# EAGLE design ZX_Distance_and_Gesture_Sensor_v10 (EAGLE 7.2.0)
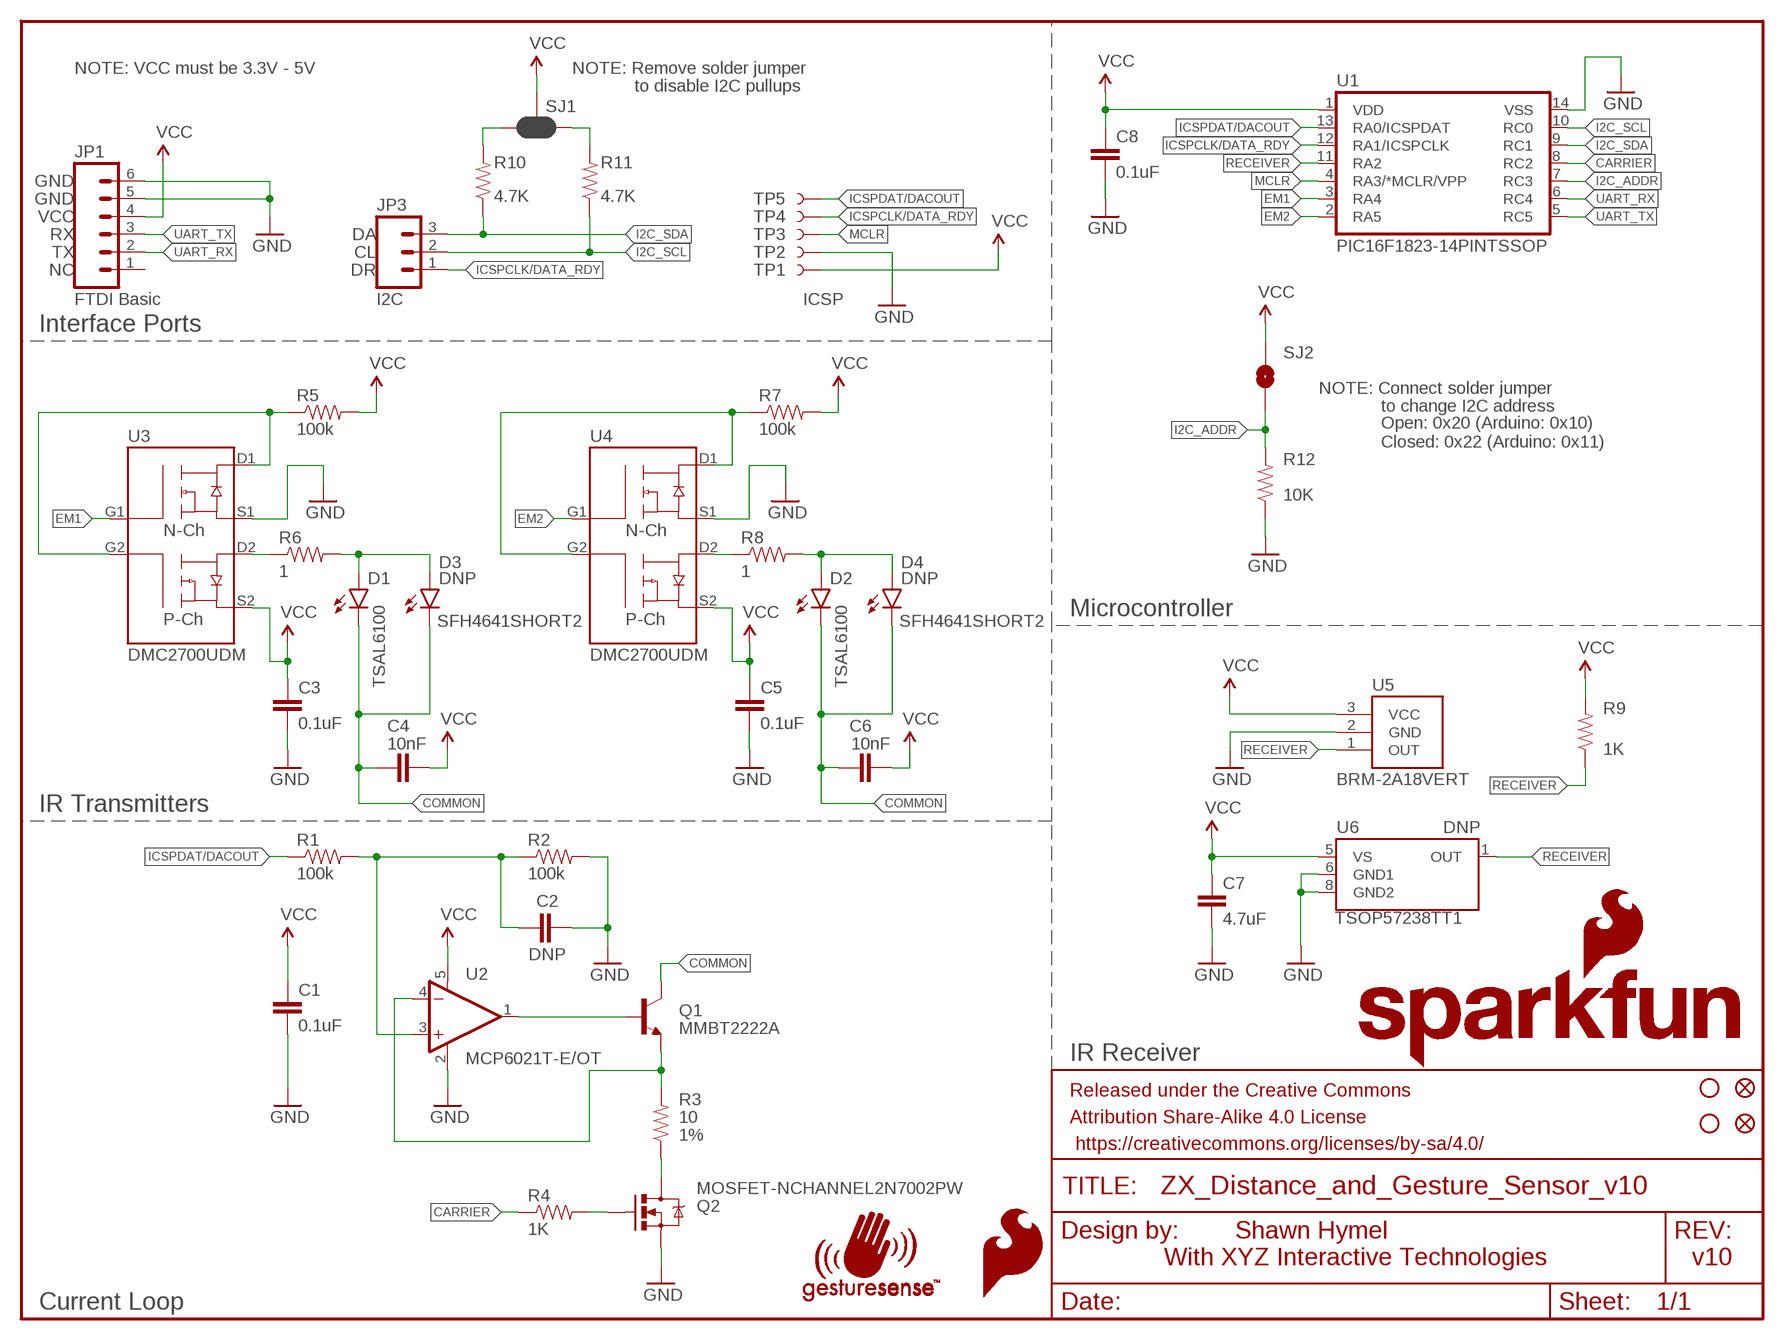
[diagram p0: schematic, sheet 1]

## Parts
C1  0.1uF  0.1UF-25V(+80/-20%)(0603)  [0603-CAP]
C2  DNP  CAP0603-CAP  [0603-CAP]
C3  0.1uF  0.1UF-25V(+80/-20%)(0603)  [0603-CAP]
C4  10nF  10NF/10000PF-50V-10%(0603)  [0603-CAP]
C5  0.1uF  0.1UF-25V(+80/-20%)(0603)  [0603-CAP]
C6  10nF  10NF/10000PF-50V-10%(0603)  [0603-CAP]
C7  4.7uF  4.7UF-6.3V-10%(0603)0603  [0603-CAP]
C8  0.1uF  0.1UF-25V(+80/-20%)(0603)  [0603-CAP]
D1  LED-IR-THRUTSAL6100  [LED5MM]
D2  LED-IR-THRUTSAL6100  [LED5MM]
D3  SFH4641SHORT2  [SFH4641-SHORT2]
D4  SFH4641SHORT2  [SFH4641-SHORT2]
FID1  FIDUCIAL1X2  [FIDUCIAL-1X2]
FID2  FIDUCIAL1X2  [FIDUCIAL-1X2]
FRAME1  FRAME-LETTER  [CREATIVE_COMMONS]
JP1  M06NO_SILK_FEMALE_PTH  [1X06_NO_SILK]
JP3  M031X03_NO_SILK  [1X03_NO_SILK]
LOGO1  SFE_LOGO_FLAME.1_INCH  [SFE_LOGO_FLAME_.1]
Q1  MMBT2222A  TRANSISTOR_NPNMMBT2222A  [SOT23-3]
Q2  MOSFET-NCHANNEL2N7002PW  [SOT323]
R1  100k  100KOHM-1/10W-1%(0603)  [0603-RES]
R2  100k  100KOHM-1/10W-1%(0603)  [0603-RES]
R3  10  10OHM-1/10W-1%(0603)SMD  [0603-RES]
R4  1K  1KOHM-1/10W-1%(0603)  [0603-RES]
R5  100k  100KOHM-1/10W-1%(0603)  [0603-RES]
R6  1  1OHM1/10W1%(0603)  [0603-RES]
R7  100k  100KOHM-1/10W-1%(0603)  [0603-RES]
R8  1  1OHM1/10W1%(0603)  [0603-RES]
R9  1K  1KOHM-1/10W-1%(0603)  [0603-RES]
R10  4.7K  4.7KOHM-1/10W-1%(0603)  [0603-RES]
R11  4.7K  4.7KOHM-1/10W-1%(0603)  [0603-RES]
R12  10K  10KOHM-1/10W-1%(0603)0603  [0603-RES]
SJ1  JUMPER-PAD-3-NC_BY_PASTE  [PAD-JUMPER-3-NC_BY_PASTE_YES_SILK_FULL_BOX]
SJ2  JUMPER-PAD-2-NOYES_SILK  [PAD-JUMPER-2-NO_YES_SILK]
STANDOFF1  STAND-OFF  [STAND-OFF]
STANDOFF2  STAND-OFF  [STAND-OFF]
TP1  TEST-POINT3X4  [PAD.03X.04]
TP2  TEST-POINT3X4  [PAD.03X.04]
TP3  TEST-POINT3X4  [PAD.03X.04]
TP4  TEST-POINT3X4  [PAD.03X.04]
TP5  TEST-POINT3X4  [PAD.03X.04]
U1  PIC16F1823-14PINTSSOP  [TSSOP14]
U2  MCP6021T-E/OT  [SOT23-5]
U3  DMC2700UDM  [SOT26]
U4  DMC2700UDM  [SOT26]
U5  BRM-2A18VERT  [BRM-2508_VERT]
U6  TSOP57238TT1  [TSOP572]
U$5  SFE_LOGO_NAME_FLAME.1_INCH  [SFE_LOGO_NAME_FLAME_.1]
U$6  GESTURESENSE_LOGOSTEXT  [GESTURESENSE_TEXT]

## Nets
CARRIER: R4.1 U1.8(RC2)
COMMON: C4.1 C6.1 D1.K(C) D2.K(C) D3.C D4.C Q1.3(C)
EM1: U1.3(RA4) U3.G1
EM2: U1.2(RA5) U4.G1
GND: C1.2 C2.2 C3.2 C5.2 C7.2 C8.2 JP1.5 JP1.6 Q2.2(S) R2.2 R12.1 TP2.P$1 U1.14(VSS) U2.2(V-) U3.S1 U4.S1 U5.2(GND) U6.6(GND1) U6.8(GND2)
I2C_ADDR: R12.2 SJ2.1 U1.7(RC3)
I2C_SCL: JP3.2 R11.1 U1.10(RC0)
I2C_SDA: JP3.3 R10.1 U1.9(RC1)
ICSPCLK/DATA_RDY: JP3.1 TP4.P$1 U1.12(RA1/ICSPCLK)
ICSPDAT/DACOUT: R1.1 TP5.P$1 U1.13(RA0/ICSPDAT)
MCLR: TP3.P$1 U1.4(RA3/*MCLR/VPP)
N$1: C2.1 R1.2 R2.1 U2.3(+IN)
N$2: Q1.2(E) R3.2 U2.4(-IN)
N$3: Q1.1(B) U2.1(OUT)
N$4: Q2.3(D) R3.1
N$5: Q2.1(G) R4.2
N$6: R6.1 U3.D2
N$7: D1.A D3.A R6.2
N$8: R5.1 U3.D1 U3.G2
N$9: R7.1 U4.D1 U4.G2
N$10: R10.2 SJ1.3
N$11: R8.1 U4.D2
N$12: D2.A D4.A R8.2
N$13: R11.2 SJ1.1
RECEIVER: R9.1 U1.11(RA2) U5.1(OUT) U6.1(OUT)
UART_RX: JP1.2 U1.6(RC4)
UART_TX: JP1.3 U1.5(RC5)
VCC: C1.1 C3.1 C4.2 C5.1 C6.2 C7.1 C8.1 JP1.4 R5.2 R7.2 R9.2 SJ1.2 SJ2.2 TP1.P$1 U1.1(VDD) U2.5(V+) U3.S2 U4.S2 U5.3(VCC) U6.5(VS)
Unconnected: JP1.1

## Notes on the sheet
- NOTE: VCC must be 3.3V - 5V | NOTE: Remove solder jumper
- to disable I2C pullups
- GND
- GND
- VCC
- RX | DA
- TX | CL
- NC | DR
- FTDI Basic | I2C | ICSP
- Interface Ports
- NOTE: Connect solder jumper
- to change I2C address
- Open: 0x20 (Arduino: 0x10)
  Closed: 0x22 (Arduino: 0x11)
- DNP | DNP
- Microcontroller
- IR Transmitters
- IR Receiver
- With XYZ Interactive Technologies
- Current Loop

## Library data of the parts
C1 C3 C5 C8 = SparkFun-Capacitors:0.1UF-25V(+80/-20%)(0603): CAP-00810; PROD_ID: CAP-00810
C2 = SparkFun-Capacitors:CAP: Capacitor
C4 C6 = SparkFun-Capacitors:10NF/10000PF-50V-10%(0603): CAP-00867; PROD_ID: CAP-00867
C7 = SparkFun-Capacitors:4.7UF-6.3V-10%(0603): CAP-08280; PROD_ID: CAP-08280
D1 D2 = SparkFun-LED:LED-IR-THRU; PROD_ID: DIO-12058; VARIANT: TSAL6100
D3 D4 = SparkFun-LED:SFH4641; PROD_ID: DIO-11994
FID1 FID2 = SparkFun-Aesthetics:FIDUCIAL: Fiducial Alignment Points
FRAME1 = SparkFun-Aesthetics:FRAME-LETTER: Schematic Frame; DESIGNER: Shawn Hymel; VERSION: v10
JP1 = SparkFun-Connectors:M06: Header 6 Standard 6-pin 0.1" header. Use with straight break away headers (SKU : PRT-00116), right angle break away headers (PRT-00553), swiss pins (PRT-00743), machine pins (PRT-00117), and female headers (PRT-00115). Molex polarized connector foot print use with SKU : PRT-08094 with associated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; PROD_ID: CONN-08437
JP3 = SparkFun-Connectors:M03: Header 3 Standard 3-pin 0.1" header. Use with straight break away headers (SKU : PRT-00116), right angle break away headers (PRT-00553), swiss pins (PRT-00743), machine pins (PRT-00117), and female headers (PRT-00115). Molex polarized connector foot print use with SKU : PRT-08232 with associated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
LOGO1 = SparkFun-Aesthetics:SFE_LOGO_FLAME: SFE Logo, flame only
Q1 = SparkFun-DiscreteSemi:TRANSISTOR_NPN: Generic NPN BJT MMBT2222A - TRANS-08049 (SOT-23, 1A 40V) MPSA42 - TRANS-09116 (SOT-23, 500mA 300V) MMBT5088LT1G - TRANS-11160 (SOT-23, 50 mA 30V) BC547 - COM-08928 (TO-92 45V 100mA) (1.Collector 2.Base 3.Emitter) 2N3904 - COM-00521 (TO-92 40V 200mA) (1.Emitter 2.Base 3.Collector) P2N2222A -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; PROD_ID: TRANS-08049
Q2 = SparkFun-DiscreteSemi:MOSFET-NCHANNEL: Common NMOSFET Parts MFG P/NStore IDProd ID FDD8780TRANS-09984 SI7820DNTRANS-11055 FDS6630AIC-08089 2N7002PWTRANS-11151 FQP30N06L COM-10213TRANS-10060 BSS123LT1GTRANS-08345 BSS138TRANS-00830 BS170 2N7000; PROD_ID: TRANS-11151
R1 R2 R5 R7 = SparkFun-Resistors:100KOHM-1/10W-1%(0603): RES-07828; PROD_ID: RES-07828
R3 = SparkFun-Resistors:10OHM-1/10W-1%(0603): RES-12581; PROD_ID: RES-12581; TOL: 1%
R4 R9 = SparkFun-Resistors:1KOHM-1/10W-1%(0603): RES-07856; PROD_ID: RES-07856
R6 R8 = SparkFun-Resistors:1OHM1/10W1%(0603): RES-08269; PROD_ID: RES-08269
R10 R11 = SparkFun-Resistors:4.7KOHM-1/10W-1%(0603): RES-07857; PROD_ID: RES-07857
R12 = SparkFun-Resistors:10KOHM-1/10W-1%(0603): RES-00824; PROD_ID: RES-00824
SJ1 = SparkFun-Passives:JUMPER-PAD-3-NC_BY_PASTE
SJ2 = SparkFun-Passives:JUMPER-PAD-2-NO
STANDOFF1 STANDOFF2 = SparkFun-Electromechanical:STAND-OFF: #4 Stand Off
TP1-TP5 = SparkFun-Passives:TEST-POINT: Bare copper test points for troubleshooting or ICT
U1 = SparkFun-DigitalIC:PIC16F1823-14PIN; PROD_ID: IC-11992
U2 = SparkFun-AnalogIC:MCP6021: Rail-to-rail input/output op-amp with 10 MHz bandwidth.; PROD_ID: IC-12504
U3 U4 = SparkFun-DiscreteSemi:DMC2700UDM; PROD_ID: TRANS-11993
U5 = SparkFun-Sensors:BRM-2A18: BRM-2A18 IR receiver.; PROD_ID: COMP-12505
U6 = SparkFun-Sensors:TSOP57238TT1; PLACE: DNP; PROD_ID: COMP-11990
U$5 = SparkFun-Aesthetics:SFE_LOGO_NAME_FLAME: SFE Logo, name and flame
U$6 = SparkFun-Aesthetics:GESTURESENSE_LOGOS

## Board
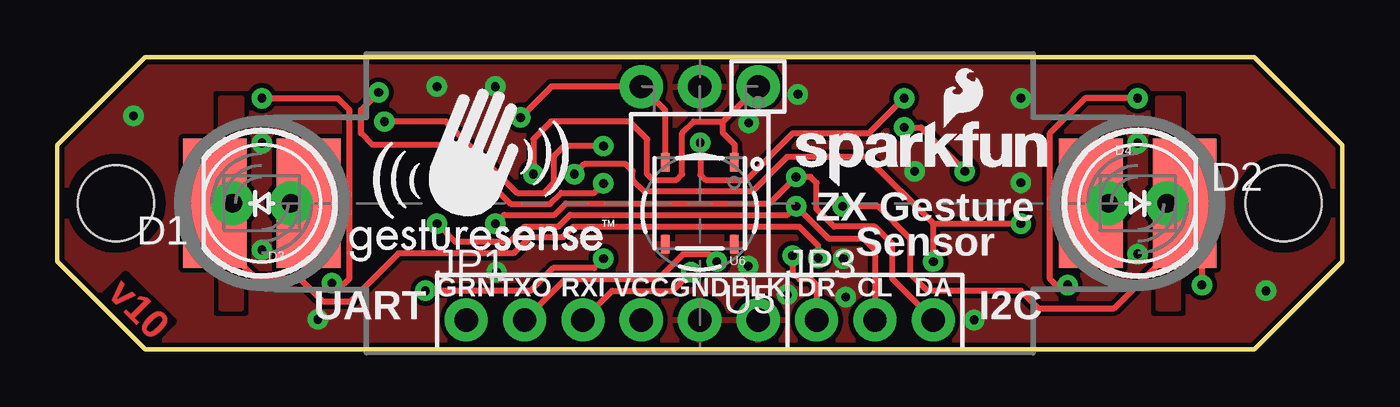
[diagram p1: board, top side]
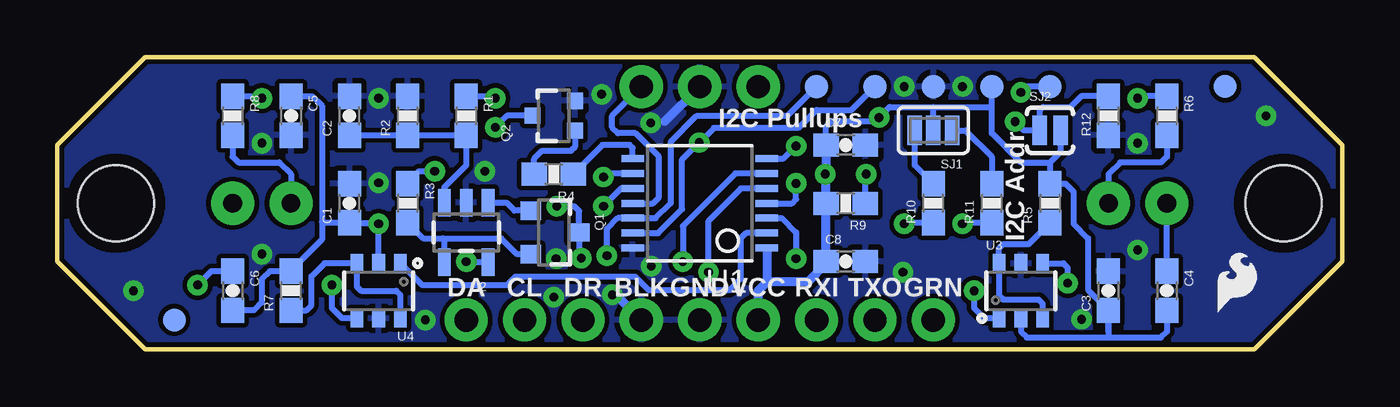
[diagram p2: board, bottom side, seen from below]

Size 55.88 x 12.7 mm. Coordinates in mm from the lower left corner, seen from the top.
Outline: 3.81,12.7 52.07,12.7 55.88,8.89 55.88,3.81 52.07,0 3.81,0 0,3.81 0,8.89 3.81,12.7
Copper layers (1*16): Top 0.035mm / dielectric 1.5mm / Bottom 0.035mm
Design rules "SparkFun-2-layer": minimum track width 7mil, minimum drill 15mil, track to track 8mil, track to pad 8mil, pad to pad 8mil, via to via 8mil, smd to smd 8mil, copper to edge 8mil, drill to drill 8mil, minimum pad ring 12mil, minimum via ring 10mil, stop-mask expansion 4mil, vias tented up to drill 20mil, thermal gap 10mil
bRestrict: 2 lines

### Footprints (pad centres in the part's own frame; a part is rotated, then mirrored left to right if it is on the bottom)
0603-CAP = smd 1.1 x 1: 1 -0.85,0; 2 0.85,0
LED5MM = drill 0.813 pad 1.88: A -1.27,0; K 1.27,0
SFH4641-SHORT2 = smd 5.62 x 2.77: A 0,-2.035; C 0,2.035
FIDUCIAL-1X2 = smd 1 x 1: 1 0,0
1X06_NO_SILK = drill 1.016 pad 1.88: 1 0,0; 2 2.54,0; 3 5.08,0; 4 7.62,0; 5 10.16,0; 6 12.7,0
1X03_NO_SILK = drill 1.016 pad 1.88: 1 0,0; 2 2.54,0; 3 5.08,0
SOT23-3 = smd 0.8 x 0.9: 1 -0.95,-1; 2 0.95,-1; 3 0,1.1
SOT323 = smd 0.7 x 0.7: 1 -0.65,-0.925; 2 0.65,-0.925; 3 0,0.925
0603-RES = smd 1.1 x 1: 1 -0.85,0; 2 0.85,0
PAD-JUMPER-3-NC_BY_PASTE_YES_SILK_FULL_BOX = smd 0.635 x 1.27: 1 -0.813,0; 2 0,0; 3 0.813,0
PAD-JUMPER-2-NO_YES_SILK = smd 0.635 x 1.27: 1 -0.45,0; 2 0.45,0
STAND-OFF = hole 3.302: 0,0
PAD.03X.04 = smd 1.016 x 1.016: P$1 0,0
TSSOP14 = smd 0.305 x 0.991: 1 -1.95,-2.918; 2 -1.3,-2.918; 3 -0.65,-2.918; 4 0,-2.918; 5 0.65,-2.918; 6 1.3,-2.918; 7 1.95,-2.918; 8 1.95,2.918; 9 1.3,2.918; 10 0.65,2.918; 11 0,2.918; 12 -0.65,2.918; 13 -1.3,2.918; 14 -1.95,2.918
SOT23-5 = smd 0.55 x 1.2: 1 -0.95,-1.3; 2 0,-1.3; 3 0.95,-1.3; 4 0.95,1.3; 5 -0.95,1.3
SOT26 = smd 0.55 x 0.8: D1 -0.95,1.2; D2 0.95,1.2; G1 -0.95,-1.2; G2 0.95,-1.2; S1 0,1.2; S2 0,-1.2
BRM-2508_VERT = drill 1.016 pad 1.88: 1 -2.54,0; 2 0,0; 3 2.54,0
TSOP572 = smd 0.35 x 0.8: 1 -1.5,-1.775; 5 1.5,-1.775; 6 1.5,1.775; 8 -1.5,1.775

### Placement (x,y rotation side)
C1  43.18,6.35 90 bottom
C2  43.18,10.16 90 bottom
C3  10.16,2.54 90 bottom
C4  7.62,2.54 270 bottom
C5  45.72,10.16 270 bottom
C6  48.26,2.54 270 bottom
C7  21.59,8.89 0 bottom
C8  21.59,3.81 0 bottom
D1  8.89,6.35 180 top
D2  46.99,6.35 0 top
D3  8.89,6.35 90 top
D4  46.99,6.35 270 top
FID1  5.08,11.43 0 bottom
FID2  50.8,1.27 0 bottom
FRAME1  not placed on the board
JP1  17.78,1.27 0 top
JP3  33.02,1.27 0 top
LOGO1  5.71,1.27 0 bottom
Q1  34.29,5.08 270 bottom
Q2  34.29,10.16 90 bottom
R1  38.1,10.16 270 bottom
R2  40.64,10.16 90 bottom
R3  40.64,6.35 270 bottom
R4  34.29,7.62 180 bottom
R5  12.7,6.35 90 bottom
R6  7.62,10.16 270 bottom
R7  45.72,2.54 90 bottom
R8  48.26,10.16 270 bottom
R9  21.59,6.35 180 bottom
R10  17.78,6.35 90 bottom
R11  15.24,6.35 90 bottom
R12  10.16,10.16 90 bottom
SJ1  17.78,9.52 180 bottom
SJ2  12.7,9.52 0 bottom
STANDOFF1  2.54,6.35 0 top
STANDOFF2  53.34,6.35 0 top
TP1  15.24,11.43 90 bottom
TP2  17.78,11.43 0 bottom
TP3  12.7,11.43 0 bottom
TP4  22.86,11.43 0 bottom
TP5  20.32,11.43 0 bottom
U1  27.94,6.35 90 bottom
U2  38.1,5.08 180 bottom
U3  13.97,2.54 0 bottom
U4  41.91,2.54 180 bottom
U5  27.94,11.43 180 top
U6  27.94,6.35 180 top
U$5  31.7,7.01 0 top
U$6  12.7,3.81 0 top

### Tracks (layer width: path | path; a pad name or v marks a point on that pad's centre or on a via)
CARRIER
  Bottom 0.254: R4.1 32.17,8.89 30.99,8.89 30.86,8.76 U1.8
COMMON  (via drill 0.38)
  Top 0.254: v33.1,3.96 33.1,4.5 32.26,5.33 22.45,5.33 22,4.88 20.55,4.88 19.84,4.17 14.83,4.17 12.75,2.08 11.53,2.08 10.57,3.05 8.64,3.05 6.86,4.83 D3.C D1.K | v34.16,6.22 35.69,6.22 37.08,4.83 37.08,3.3 37.85,2.54 41.91,2.54 42.67,1.78 45.97,1.78 49.02,4.83 | D2.K D4.C 49.02,4.83 | 49.02,4.83 49.78,4.06 v49.78,2.79
  Bottom 0.254: v33.1,3.96 33.19,4.06 Q1.3 33.19,6.01 33.4,6.22 v34.16,6.22 | C6.1 49.19,3.39 v49.78,2.79 | C4.1 D1.K
EM1  (via drill 0.38)
  Top 0.254: v16,2.54 20.57,2.54 21.57,3.53 23.34,3.53 v23.75,3.94
  Bottom 0.254: U1.3 24.37,5.7 23.75,5.08 v23.75,3.94 | U3.G1 15.56,1.34 16,1.78 v16,2.54
EM2
  Bottom 0.254: U1.2 25.94,5.05 26.16,4.83 26.16,3.05 26.65,2.56 30.15,2.56 30.73,3.15 35.97,3.15 36.32,2.79 40.01,2.79 U4.G1
GND  (via drill 0.38)
  Bottom 0.254: v34.19,3.94 34.16,3.94
  Bottom 0.381: 29.46,9.91 U5.2 | 31.75,2.54 JP1.6
  other vias: 8.89,8.97 8.89,4.32 34.29,2.26 37.29,7.75 41.91,10.92 46.99,8.97 41.91,7.24 39.88,1.27 30.05,3.61 16.51,11.43 11.33,1.3 30.07,9.86 52.58,2.54 3.3,10.16 19.05,11.43 19.1,3.35 32.21,11.1 31.75,2.36 46.99,4.14
  pour Top (isolate 0.203, rank 5): 3.81,0 52.07,0 55.88,3.81 55.88,8.89 52.07,12.7 3.81,12.7 0,8.89 0,3.81
  pour Bottom (isolate 0.203): 3.81,0 52.07,0 55.88,3.81 55.88,8.89 52.07,12.7 3.81,12.7 0,8.89 0,3.81
I2C_ADDR  (via drill 0.38)
  Top 0.254: v23.75,8.84 22.05,8.84 21.59,8.38 21.59,7.24 21.16,6.81 19.99,6.81 16.89,9.91 v14.22,9.91
  Bottom 0.254: R12.2 11.34,11.01 11.81,10.54 13.01,10.54 13.15,10.4 SJ2.1 13.84,9.52 v14.22,9.91 | U1.7 24.29,8.3 v23.75,8.84
I2C_SCL  (via drill 0.38)
  Top 0.254: JP3.2 35.56,4.32 35.05,4.83 33.53,4.83 v32.13,6.22 31.75,5.84 22.3,5.84 21.79,5.33 20.32,5.33 19.66,4.67 17.3,4.67 v16.51,5.46
  Bottom 0.254: R11.1 16.47,5.5 v16.51,5.46 | U1.10 31.35,7 v32.13,6.22
I2C_SDA  (via drill 0.38)
  Top 0.254: JP3.3 36.32,3.05 36.32,4.57 35.56,5.33 33.78,5.33 33.02,6.1 33.02,7.24 32.77,7.49 v32.13,7.49 31.18,6.54 30.99,6.35 22.12,6.35 21.62,5.84 19.43,5.84 v19.05,5.46
  Bottom 0.254: R10.1 19.01,5.5 v19.05,5.46 | U1.9 31.97,7.65 v32.13,7.49
ICSPCLK/DATA_RDY  (via drill 0.38)
  Top 0.254: v31.98,4.06 31.98,3.33 32.26,3.05 32.77,3.05 33.02,2.79 JP3.1
  Bottom 0.254: TP4.P$1 24.16,10.13 28.09,10.13 29.21,9.02 29.21,6.35 29.86,5.7 U1.12 31.51,5.7 31.98,5.23 v31.98,4.06
ICSPDAT/DACOUT  (via drill 0.38)
  Top 0.254: v36.83,10.92 35.31,9.4 32,9.4 29.97,7.37 28.19,7.37 27.96,7.59 v27.96,8.99
  Bottom 0.254: R1.1 36.92,11.01 v36.83,10.92 | TP5.P$1 21.34,10.41 22.86,10.41 23.65,9.63 27.33,9.63 v27.96,8.99 28.7,8.25 28.7,6.1 29.75,5.05 U1.13
MCLR  (via drill 0.38)
  Top 0.254: v23.75,7.21 23.34,6.81 21.92,6.81 21.44,6.32 19.71,6.32 17.15,8.89 13.72,8.89 13.21,9.4 13.21,10.41 v13.97,11.18
  Bottom 0.254: U1.4 23.93,6.35 23.75,6.53 v23.75,7.21 | TP3.P$1 13.72,11.43 v13.97,11.18
N$1
  Bottom 0.254: C2.1 R2.1 R1.2 38.1,8 39.05,7.05 U2.3
N$2
  Bottom 0.254: Q1.2 35.88,4.13 36.58,4.83 39.12,4.83 | 39.12,4.83 39.97,4.83 R3.2 | U2.4 39.05,4.76 39.12,4.83
N$3
  Bottom 0.254: U2.1 36.35,6.38 36,6.03 Q1.1
N$4  (via drill 0.38)
  Top 0.254: v36.83,9.65 37.57,9.65 v39.47,7.75
  Bottom 0.254: Q2.3 36.32,10.16 v36.83,9.65 | R3.1 40.64,7.26 40.16,7.75 v39.47,7.75
N$5
  Bottom 0.254: Q2.1 33.37,8.8 33.53,8.64 34.8,8.64 35.14,8.29 R4.2
N$6  (via drill 0.38)
  Top 0.254: v8.89,10.92 12.19,10.92 12.7,10.41 12.7,3.07 12.5,2.87 v11.94,2.87
  Bottom 0.254: R6.1 8.8,11.01 v8.89,10.92 | U3.D2 12.12,3.74 11.94,3.56 v11.94,2.87
N$7
  Top 0.254: D3.A D1.A
  Bottom 0.254: R6.2 7.62,8.38 7.87,8.13 9.65,8.13 10.16,7.62 D1.A
N$8
  Bottom 0.254: R5.1 13.63,4.57 14.73,4.57 14.92,4.38 U3.D1 14.92,2.35 14.73,2.16 13.21,2.16 13.02,1.97 U3.G2
N$9
  Bottom 0.254: U4.D1 40.96,2.35 41.15,2.54 42.67,2.54 42.86,2.73 U4.G2 44.27,3.74 44.83,3.17 44.83,1.9 45.05,1.69 R7.1
N$10
  Bottom 0.254: SJ1.3 18.59,8.01 R10.2
N$11  (via drill 0.38)
  Top 0.254: v46.99,10.92 44.7,10.92 43.18,9.4 43.18,3.05 43.43,2.79 v43.94,2.79
  Bottom 0.254: U4.D2 43.5,1.34 43.94,1.78 v43.94,2.79 | R8.1 47.08,11.01 v46.99,10.92
N$12
  Top 0.254: D4.A D2.A
  Bottom 0.254: R8.2 48.26,8.38 48.01,8.13 46.23,8.13 45.72,7.62 D2.A
N$13
  Bottom 0.254: SJ1.1 16.38,9.52 15.24,8.38 R11.2
N$15
  pour Top (isolate 0.305): 7.11,10.92 8,10.92 8,9.65 7.11,9.65
N$16
  pour Top (isolate 0.305): 48.77,3.05 47.88,3.05 47.88,1.78 48.77,1.78
N$17
  pour Top (isolate 0.305): 48.77,9.65 47.88,9.65 47.88,10.92 48.77,10.92
N$18
  pour Top (isolate 0.305): 7.11,3.05 7.11,1.78 8,1.78 8,3.05
RECEIVER  (via drill 0.38)
  Top 0.254: v20.7,7.62 20.7,9.14 21.46,9.91 24.89,9.91 25.65,9.14 25.65,7.62 25.91,7.37 26.92,7.37 27.18,7.62 27.18,9.4 27.69,9.91 28.96,9.91 | U6.1 29.46,8.15 29.46,8.89 28.96,9.4 28.96,9.91 | 28.96,9.91 U5.1
  Bottom 0.254: R9.1 20.74,7.58 v20.7,7.62 | U1.11 29.97,6.35 29.72,6.6 29.72,8.38 30.73,9.4 31.5,9.4 31.75,9.65 31.75,10.16 U5.1
UART_RX  (via drill 0.38)
  Top 0.254: JP1.2 22.1,3.05 26.14,3.05 27.23,4.14 28.35,4.14 v28.68,3.81
  Bottom 0.254: U1.6 26.39,7.65 28.68,5.36 v28.68,3.81
UART_TX  (via drill 0.38)
  Top 0.254: JP1.3 24.13,2.54 26.75,2.54 v27.56,3.35
  Bottom 0.254: U1.5 26.15,7 27.56,5.59 v27.56,3.35
VCC  (via drill 0.38)
  Top 0.254: U6.5 26.44,10.39 U5.3 21.49,11.43 v20.14,10.08 | v38.1,3.81 38.1,5.46 | 38.1,5.46 v41.91,5.46 | v22.48,7.62 22.91,8.05 24.71,8.05 25.02,7.75 25.02,7.37 25.53,6.86 30.23,6.86 31.75,8.38 35.18,8.38 38.1,5.46
  Bottom 0.254: C5.1 44.79,11.01 44.37,10.59 44.37,5.54 | 15.24,10.54 TP1.P$1 | 12.7,8.13 R5.2 12.03,7.2 11.68,6.86 11.68,5.46 11.05,4.83 11.05,2.58 C3.1 | SJ1.2 17.78,10.54 | 17.78,10.54 19.69,10.54 v20.14,10.08 20.32,9.91 22.23,9.91 22.44,9.69 C7.1 | 17.78,10.54 15.24,10.54 | U3.S2 13.97,0.76 13.72,0.51 10.16,0.51 | 10.16,0.51 7.87,0.51 7.62,0.76 C4.2 | SJ2.2 12.25,8.58 12.7,8.13 | 12.7,8.13 13.97,8.13 15.24,9.4 15.24,10.54 | U1.1 25.02,4.35 25.02,4.34 | U2.5 38.07,3.78 v38.1,3.81 | U4.S2 v41.91,5.46 41.95,5.5 C1.1 44.34,5.5 44.37,5.54 | 44.37,5.54 44.37,4.77 45.72,3.43 R7.2 46.65,3.39 46.99,3.05 46.99,2.03 47.33,1.69 C6.2 | 10.16,0.76 C3.1 | C3.1 10.16,0.51
  Bottom 0.381: 25.02,2.92 25.4,2.54 JP1.4 | 25.02,2.92 23.24,2.92 22.44,3.72 C8.1 R9.2 22.44,7.58 v22.48,7.62 22.44,7.66 C7.1 | 25.02,4.34 25.02,2.92

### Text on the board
Top: v10
tPlace: ZX Gesture | Sensor | UART | GRN | TXO | RXI | VCC | GND | BLK | DR | CL | DA | I2C
bPlace: I2C Pullups | I2C Addr | GRN | TXO | RXI | VCC | GND | BLK | DR | CL | DA
tDocu: Shawn Hymel (SparkFun Electronics) / with XYZ Interactive Technologies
